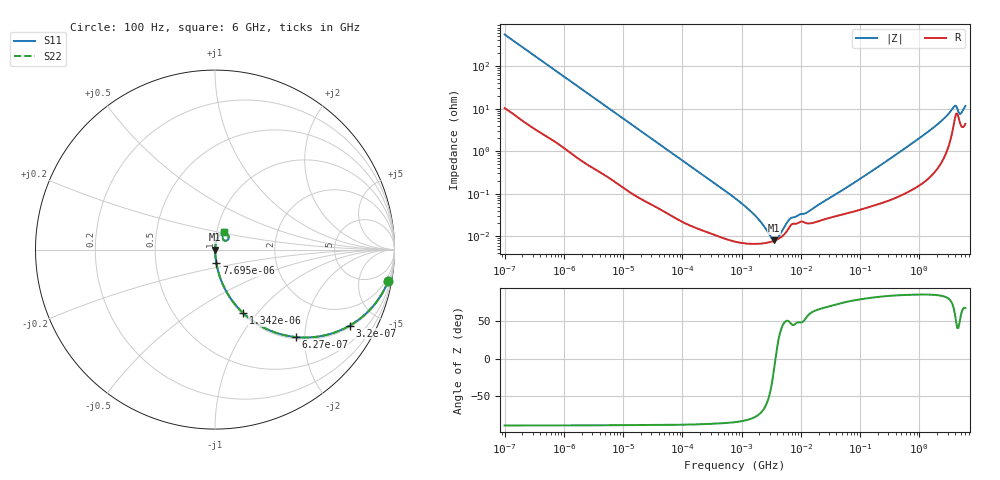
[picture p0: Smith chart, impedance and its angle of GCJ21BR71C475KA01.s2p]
!Murata Part Number: GCJ21BR71C475KA01
!These Parameters are Measured in Series Mode Connection
!Data Generated on Mar 13, 2026
!  o--ll--o
!Port1  Port2
!  o------o
!Operation Temp=25[degC], DC Bias Voltage=0[V]
!Freq. Start=100[Hz] Stop=6[GHz] 401[Steps]
# Hz S RI R 50
!Freq.(Hz) S11(Real) S11(Imag) S21(Real) S21(Imag) S12(Real) S12(Imag) S22(Real) S22(Imag)
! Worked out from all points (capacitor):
!   401 points, 100 Hz to 6 GHz, reference 50 ohm
!   read as one part in series: C = 2.87 uF near 109 Hz
!   lowest |Z| = 8.02 mohm at 3.55 MHz (marker M1)
!   series resonance near 3.732 MHz, so ESL is about 630 pH
!   S11 on the Smith chart (normalised r, x): 100 Hz: 1, -11; 320 Hz: 1.07, -3.50; 627 Hz: 1.04, -1.80; 1.342 kHz: 1.02, -0.85; 7.695 kHz: 1.00, -0.15; 6 GHz: 1.09, +0.21
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100  0.9652 -0.1741  0.0348 0.1741  0.0348 0.1741  0.9652 -0.1741
196  0.8858 -0.3089  0.1142 0.3089  0.1142 0.3089  0.8858 -0.3089
320  0.7497 -0.4238  0.2503 0.4238  0.2503 0.4238  0.7497 -0.4238
627  0.4495 -0.4872  0.5505 0.4872  0.5505 0.4872  0.4495 -0.4872
1342  0.1585 -0.3551  0.8415 0.3551  0.8415 0.3551  0.1585 -0.3551
2008  0.0801 -0.2614  0.9199 0.2614  0.9199 0.2614  0.0801 -0.2614
3759  0.0263 -0.1493  0.9737 0.1493  0.9737 0.1493  0.0263 -0.1493
7695  0.0075 -0.0753  0.9925 0.0753  0.9925 0.0753  0.0075 -0.0753
40335  0.000665 -0.0148  0.9993 0.0148  0.9993 0.0148  0.000665 -0.0148
774597  7.52e-05 -0.000783  0.9999 0.000783  0.9999 0.000783  7.52e-05 -0.000783
1734173  6.61e-05 -0.000289  0.9999 0.000289  0.9999 0.000289  6.61e-05 -0.000289
2967816  7.24e-05 -7.97e-05  0.9999 7.97e-05  0.9999 7.97e-05  7.24e-05 -7.97e-05
3549919  7.83e-05 -1.73e-05  0.9999 1.73e-05  0.9999 1.73e-05  7.83e-05 -1.73e-05
4440638  9.13e-05 6.13e-05  0.9999 -6.13e-05  0.9999 -6.13e-05  9.13e-05 6.13e-05
6644369  0.000175 0.000194  0.9998 -0.000194  0.9998 -0.000194  0.000175 0.000194
1.243624e7  0.000203 0.000291  0.9998 -0.000291  0.9998 -0.000291  0.000203 0.000291
1.555665e7  0.000204 0.000387  0.9998 -0.000387  0.9998 -0.000387  0.000204 0.000387
3.124326e8  0.000736 0.00644  0.9993 -0.00644  0.9993 -0.00644  0.000736 0.00644
1.791126e9  0.00447 0.0367  0.9955 -0.0367  0.9955 -0.0367  0.00447 0.0367
3.8344e9  0.051 0.092  0.949 -0.092  0.949 -0.092  0.051 0.092
5.016141e9  0.0429 0.0591  0.9571 -0.0591  0.9571 -0.0591  0.0429 0.0591
6e9  0.0519 0.0972  0.9481 -0.0972  0.9481 -0.0972  0.0519 0.0972
